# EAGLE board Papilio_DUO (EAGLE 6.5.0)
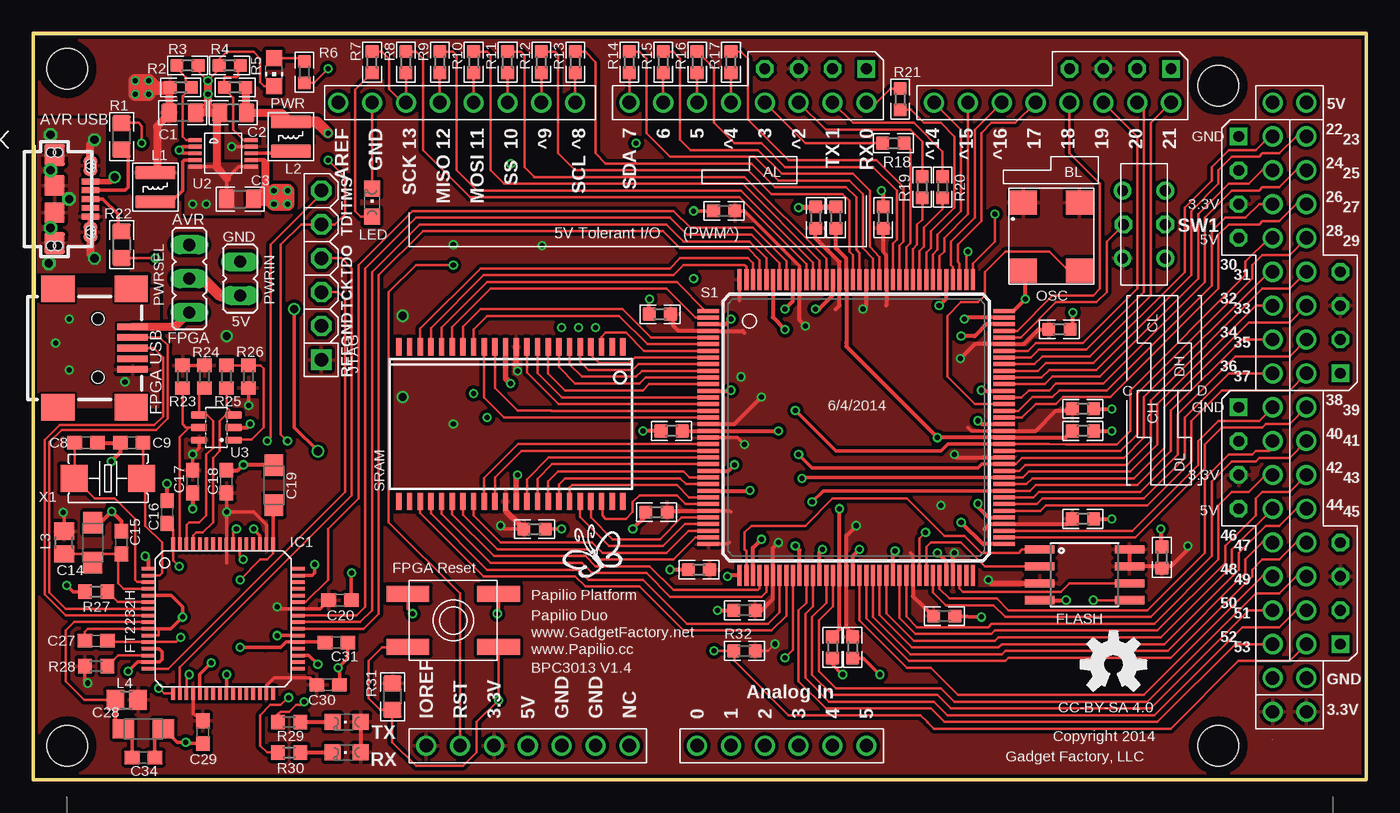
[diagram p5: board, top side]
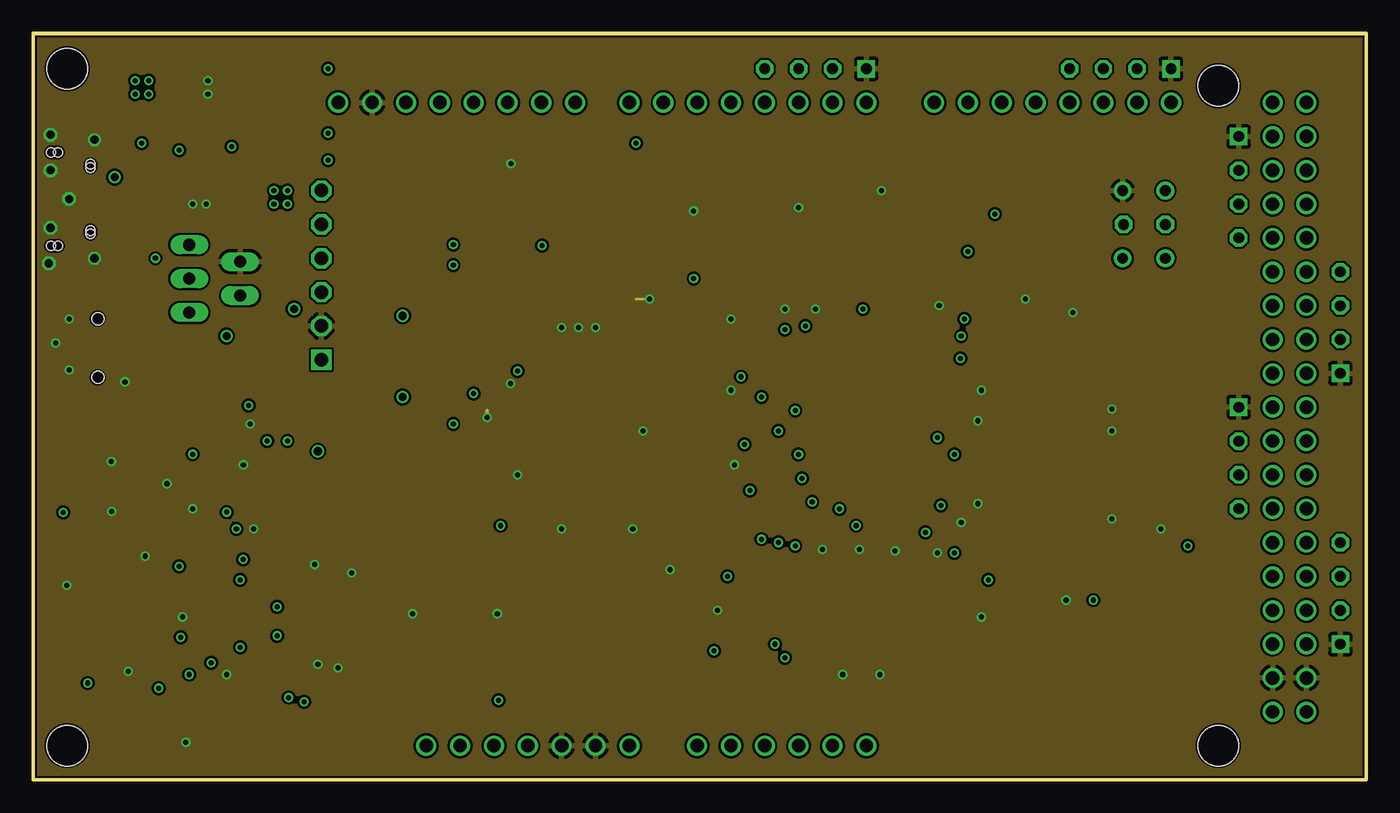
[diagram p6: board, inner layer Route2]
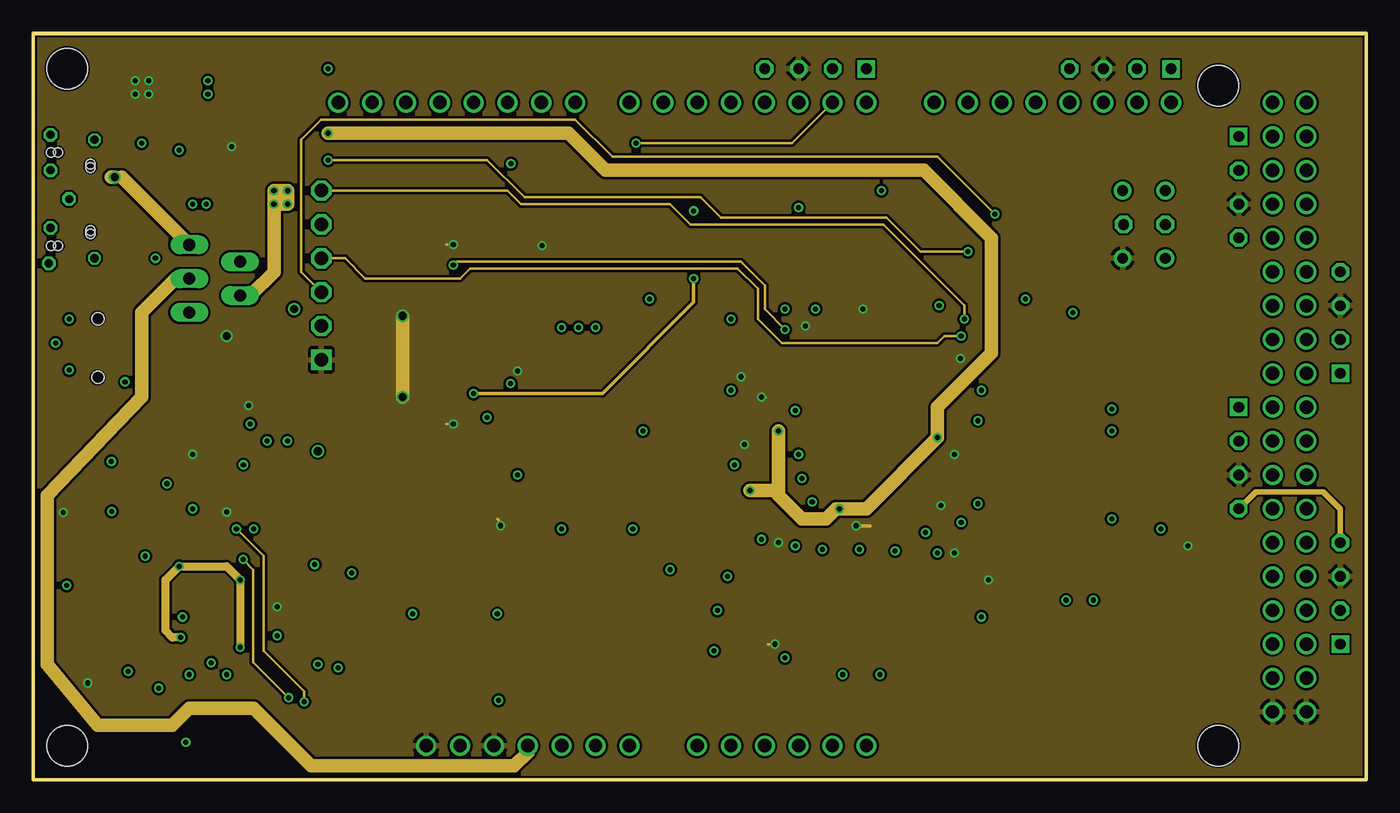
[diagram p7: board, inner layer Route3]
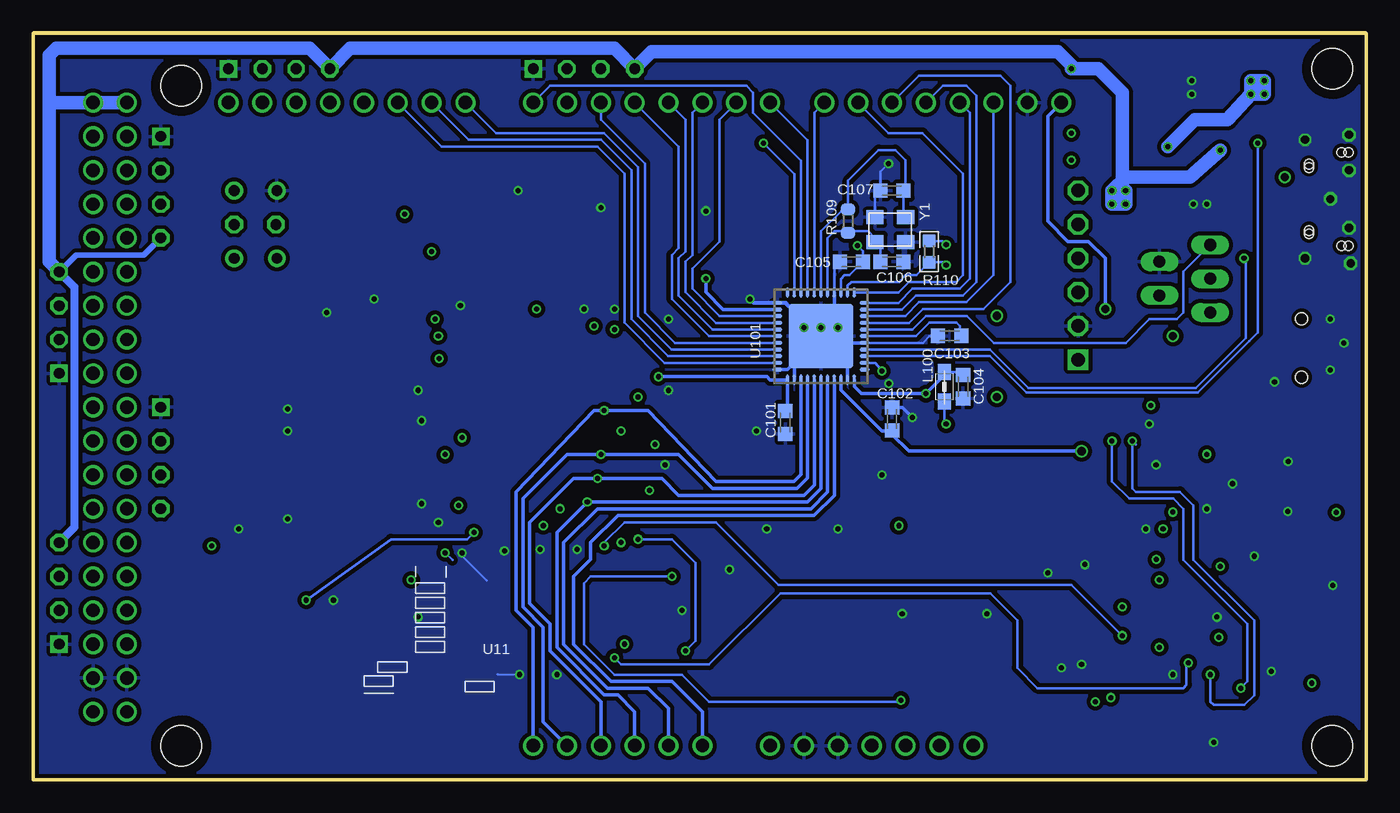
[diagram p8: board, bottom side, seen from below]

Size 100 x 56 mm. Coordinates in mm from the lower left corner, seen from the top.
Outline: 0,56 100,56 100,0 0,0 0,56
Outline: 0,56 56,56
Copper layers (1*2+3*16): Top 0.035mm / dielectric 1.5mm / Route2 0.035mm / dielectric 0.15mm / Route3 0.035mm / dielectric 0.2mm / Bottom 0.035mm
Design rules "hackvana *": minimum track width 6mil, minimum drill 0.3mm, track to track 6mil, track to pad 6mil, pad to pad 6mil, via to via 6mil, smd to smd 0mil, copper to edge 6mil, drill to drill 6mil, minimum pad ring 10mil, minimum via ring 6mil, stop-mask expansion 2mil, vias tented up to drill 100mil, thermal gap 10mil
Net classes: 0 default: width 0.178 mm, drill 0.381 mm, clearance 0.178 mm; 1 Power: width 0.254 mm, drill 0.381 mm, clearance 0.178 mm; 2 gnd: width 0.254 mm, drill 0.61 mm, clearance 0.254 mm; 3 usbvcc: width 0.254 mm, drill 0.61 mm, clearance 0.254 mm; 4 aref: width 0.254 mm, drill 0.61 mm, clearance 0.254 mm

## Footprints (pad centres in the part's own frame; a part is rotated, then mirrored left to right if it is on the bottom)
CON2_USB_MICRO_B_AT = smd 0.406 x 1.346: P1 -1.321,2.692; P2 -0.66,2.692; P3 0,2.692; P4 0.66,2.692; P5 1.321,2.692 | smd 1.651 x 1.549: S1 -3.302,0; S2 3.302,0 | smd 1.524 x 1.016: S3 -2.489,2.692; S4 2.489,2.692 | smd 1.524 x 1.524: S5 -1.016,0; S6 1.016,0 | hole 0.7: -3.505,0.254; -3.505,-0.254; 3.505,0.254; 3.505,-0.254; -2.616,2.692; -2.362,2.692; 2.362,2.692; 2.616,2.692
0805 = smd 1.2 x 1.4: 1 -1,0; 2 1,0
0603 = smd 1 x 1: 1 -0.8,0; 2 0.8,0
C603 = smd 1.1 x 1: 1 -0.85,0; 2 0.85,0
SMC_A = smd 1.6 x 1.4: + -1.5,0; - 1.5,0
C0603K = smd 1.05 x 1.08: 1 -0.875,0; 2 0.875,0
SO08-EIAJ = smd 0.61 x 2.21: 1 -1.905,-3.378; 2 -0.635,-3.378; 3 0.635,-3.378; 4 1.905,-3.378; 5 1.905,3.353; 6 0.635,3.353; 7 -0.635,3.353; 8 -1.905,3.353
CONN_USB_MINI-B = smd 2 x 2.5: BODY@1 -4.45,2.5; BODY@2 4.45,2.5; BODY@3 4.45,-3; BODY@4 -4.45,-3 | smd 0.5 x 2.3: D+ 0,2.6; D- -0.8,2.6; GND 1.6,2.6; ID 0.8,2.6; VUSB -1.6,2.6 | hole 0.9: -2.2,0; 2.2,0
LQFP64 = smd 1 x 0.27: 1 -5.6,3.75; 2 -5.6,3.25; 3 -5.6,2.75; 4 -5.6,2.25; 5 -5.6,1.75; 6 -5.6,1.25; 7 -5.6,0.75; 8 -5.6,0.25; 9 -5.6,-0.25; 10 -5.6,-0.75; 11 -5.6,-1.25; 12 -5.6,-1.75; 13 -5.6,-2.25; 14 -5.6,-2.75; 15 -5.6,-3.25; 16 -5.6,-3.75; 33 5.6,-3.75; 34 5.6,-3.25; 35 5.6,-2.75; 36 5.6,-2.25; 37 5.6,-1.75; 38 5.6,-1.25; 39 5.6,-0.75; 40 5.6,-0.25; 41 5.6,0.25; 42 5.6,0.75; 43 5.6,1.25; 44 5.6,1.75; 45 5.6,2.25; 46 5.6,2.75; 47 5.6,3.25; 48 5.6,3.75 | smd 0.27 x 1: 17 -3.75,-5.6; 18 -3.25,-5.6; 19 -2.75,-5.6; 20 -2.25,-5.6; 21 -1.75,-5.6; 22 -1.25,-5.6; 23 -0.75,-5.6; 24 -0.25,-5.6; 25 0.25,-5.6; 26 0.75,-5.6; 27 1.25,-5.6; 28 1.75,-5.6; 29 2.25,-5.6; 30 2.75,-5.6; 31 3.25,-5.6; 32 3.75,-5.6; 49 3.75,5.6; 50 3.25,5.6; 51 2.75,5.6; 52 2.25,5.6; 53 1.75,5.6; 54 1.25,5.6; 55 0.75,5.6; 56 0.25,5.6; 57 -0.25,5.6; 58 -0.75,5.6; 59 -1.25,5.6; 60 -1.75,5.6; 61 -2.25,5.6; 62 -2.75,5.6; 63 -3.25,5.6; 64 -3.75,5.6
VLS3015 = smd 3 x 1: 1 0,1.1; 2 0,-1.1
FB603 = smd 1.3 x 1.5: 1 -0.85,0; 2 0.85,0
0805' = smd 1.2 x 1: 1 -1.1,0; 2 1.1,0
CHIPLED_0805 = smd 1.2 x 1.2: A 0,-1.05; C 0,1.05
OSC1 = smd 1.8 x 2: 1@1 0,0; 2@2 5.08,0; 3@3 5.08,4.2; 4@4 0,4.2
CHIP-LED0805 = smd 1.2 x 1.2: A 0,-1.05; C 0,1.05
JP1 = drill 0.914 long: 1 0,-1.27; 2 0,1.27
JP2 = drill 0.914 long: 1 -2.54,0; 2 0,0; 3 2.54,0
R603 = smd 1 x 1.1: 1 -0.85,0; 2 0.85,0
R0603-ROUND = smd 0.898 x 1.1: 1 -0.889,0; 2 0.889,0
LED-805 = smd 1.2 x 1.2: A 0,-1.05; C 0,1.05
TQ144 = smd 1.6 x 0.3: 1 -11.1,8.75; 2 -11.1,8.25; 3 -11.1,7.75; 4 -11.1,7.25; 5 -11.1,6.75; 6 -11.1,6.25; 7 -11.1,5.75; 8 -11.1,5.25; 9 -11.1,4.75; 10 -11.1,4.25; 11 -11.1,3.75; 12 -11.1,3.25; 13 -11.1,2.75; 14 -11.1,2.25; 15 -11.1,1.75; 16 -11.1,1.25; 17 -11.1,0.75; 18 -11.1,0.25; 19 -11.1,-0.25; 20 -11.1,-0.75; 21 -11.1,-1.25; 22 -11.1,-1.75; 23 -11.1,-2.25; 24 -11.1,-2.75; 25 -11.1,-3.25; 26 -11.1,-3.75; 27 -11.1,-4.25; 28 -11.1,-4.75; 29 -11.1,-5.25; 30 -11.1,-5.75; 31 -11.1,-6.25; 32 -11.1,-6.75; 33 -11.1,-7.25; 34 -11.1,-7.75; 35 -11.1,-8.25; 36 -11.1,-8.75; 73 11.1,-8.75; 74 11.1,-8.25; 75 11.1,-7.75; 76 11.1,-7.25; 77 11.1,-6.75; 78 11.1,-6.25; 79 11.1,-5.75; 80 11.1,-5.25; 81 11.1,-4.75; 82 11.1,-4.25; 83 11.1,-3.75; 84 11.1,-3.25; 85 11.1,-2.75; 86 11.1,-2.25; 87 11.1,-1.75; 88 11.1,-1.25; 89 11.1,-0.75; 90 11.1,-0.25; 91 11.1,0.25; 92 11.1,0.75; 93 11.1,1.25; 94 11.1,1.75; 95 11.1,2.25; 96 11.1,2.75; 97 11.1,3.25; 98 11.1,3.75; 99 11.1,4.25; 100 11.1,4.75; 101 11.1,5.25; 102 11.1,5.75; 103 11.1,6.25; 104 11.1,6.75; 105 11.1,7.25; 106 11.1,7.75; 107 11.1,8.25; 108 11.1,8.75 | smd 0.3 x 1.6: 37 -8.75,-11.1; 38 -8.25,-11.1; 39 -7.75,-11.1; 40 -7.25,-11.1; 41 -6.75,-11.1; 42 -6.25,-11.1; 43 -5.75,-11.1; 44 -5.25,-11.1; 45 -4.75,-11.1; 46 -4.25,-11.1; 47 -3.75,-11.1; 48 -3.25,-11.1; 49 -2.75,-11.1; 50 -2.25,-11.1; 51 -1.75,-11.1; 52 -1.25,-11.1; 53 -0.75,-11.1; 54 -0.25,-11.1; 55 0.25,-11.1; 56 0.75,-11.1; 57 1.25,-11.1; 58 1.75,-11.1; 59 2.25,-11.1; 60 2.75,-11.1; 61 3.25,-11.1; 62 3.75,-11.1; 63 4.25,-11.1; 64 4.75,-11.1; 65 5.25,-11.1; 66 5.75,-11.1; 67 6.25,-11.1; 68 6.75,-11.1; 69 7.25,-11.1; 70 7.75,-11.1; 71 8.25,-11.1; 72 8.75,-11.1; 109 8.75,11.1; 110 8.25,11.1; 111 7.75,11.1; 112 7.25,11.1; 113 6.75,11.1; 114 6.25,11.1; 115 5.75,11.1; 116 5.25,11.1; 117 4.75,11.1; 118 4.25,11.1; 119 3.75,11.1; 120 3.25,11.1; 121 2.75,11.1; 122 2.25,11.1; 123 1.75,11.1; 124 1.25,11.1; 125 0.75,11.1; 126 0.25,11.1; 127 -0.25,11.1; 128 -0.75,11.1; 129 -1.25,11.1; 130 -1.75,11.1; 131 -2.25,11.1; 132 -2.75,11.1; 133 -3.25,11.1; 134 -3.75,11.1; 135 -4.25,11.1; 136 -4.75,11.1; 137 -5.25,11.1; 138 -5.75,11.1; 139 -6.25,11.1; 140 -6.75,11.1; 141 -7.25,11.1; 142 -7.75,11.1; 143 -8.25,11.1; 144 -8.75,11.1
TSOP44-II = smd 0.4 x 1.3: 1 -8.4,-5.8; 2 -7.6,-5.8; 3 -6.8,-5.8; 4 -6,-5.8; 5 -5.2,-5.8; 6 -4.4,-5.8; 7 -3.6,-5.8; 8 -2.8,-5.8; 9 -2,-5.8; 10 -1.2,-5.8; 11 -0.4,-5.8; 12 0.4,-5.8; 13 1.2,-5.8; 14 2,-5.8; 15 2.8,-5.8; 16 3.6,-5.8; 17 4.4,-5.8; 18 5.2,-5.8; 19 6,-5.8; 20 6.8,-5.8; 21 7.6,-5.8; 22 8.4,-5.8; 23 8.4,5.8; 24 7.6,5.8; 25 6.8,5.8; 26 6,5.8; 27 5.2,5.8; 28 4.4,5.8; 29 3.6,5.8; 30 2.8,5.8; 31 2,5.8; 32 1.2,5.8; 33 0.4,5.8; 34 -0.4,5.8; 35 -1.2,5.8; 36 -2,5.8; 37 -2.8,5.8; 38 -3.6,5.8; 39 -4.4,5.8; 40 -5.2,5.8; 41 -6,5.8; 42 -6.8,5.8; 43 -7.6,5.8; 44 -8.4,5.8
6P-2CH-2.54-9.1X3.5X3.2+2H = drill 0.813 pad 1.27: CH1A -2.54,-1.6; CH1B 2.54,-1.6; CH2A -2.54,1.6; CH2B 2.54,1.6 | drill 0.813 pad 1.27 octagon: COM1 0,-1.6; COM2 0,1.524
EVQ-Q2 = smd 3.2 x 1.2: A -3.4,-2; A' 3.4,-2; B -3.4,2; B' 3.4,2
ARDUINO_MEGA_SHIELD = drill 1 pad 1.422: 3.3V 50.8,26.67; 3V3@1 48.26,85.09; 3V3@2 48.26,87.63; 5V@0 50.8,29.21; 5V@1 2.54,85.09; 5V@2 2.54,87.63; A0 50.8,41.91; A1 50.8,44.45; A2 50.8,46.99; A3 50.8,49.53; A4 50.8,52.07; A5 50.8,54.61; AREF 2.54,14.986; D2 2.54,49.53; D3 2.54,46.99; D4 2.54,44.45; D5 2.54,41.91; D6 2.54,39.37; D7 2.54,36.83; D8 2.54,32.766; D9 2.54,30.226; D10 2.54,27.686; D11 2.54,25.146; D12 2.54,22.606; D13 2.54,20.066; D14 2.54,59.69; D15 2.54,62.23; D16 2.54,64.77; D17 2.54,67.31; D18 2.54,69.85; D19 2.54,72.39; D20 2.54,74.93; D21 2.54,77.47; D22 5.08,85.09; D23 5.08,87.63; D24 7.62,85.09; D25 7.62,87.63; D26 10.16,85.09; D27 10.16,87.63; D28 12.7,85.09; D29 12.7,87.63; D30 15.24,85.09; D31 15.24,87.63; D32 17.78,85.09; D33 17.78,87.63; D34 20.32,85.09; D35 20.32,87.63; D36 22.86,85.09; D37 22.86,87.63; D38 25.4,85.09; D39 25.4,87.63; D40 27.94,85.09; D41 27.94,87.63; D42 30.48,85.09; D43 30.48,87.63; D44 33.02,85.09; D45 33.02,87.63; D46 35.56,85.09; D47 35.56,87.63; D48 38.1,85.09; D49 38.1,87.63; D50 40.64,85.09; D51 40.64,87.63; D52 43.18,85.09; D53 43.18,87.63; GND@0 50.8,31.75; GND@1 50.8,34.29; GND@2 2.54,17.526; GND@3 45.72,85.09; GND@4 45.72,87.63; IOREF 50.8,21.59; RES 50.8,24.13; RX 2.54,54.61; TX 2.54,52.07; VIN 50.8,36.83
MSOP10 = smd 0.28 x 1: 1 -1,-2.1; 2 -0.5,-2.1; 3 0,-2.1; 4 0.5,-2.1; 5 1,-2.1; 6 1,2.1; 7 0.5,2.1; 8 0,2.1; 9 -0.5,2.1; 10 -1,2.1
SOT23-6 = smd 0.55 x 1.2: 1 -0.95,-1.3; 2 0,-1.3; 3 0.95,-1.3; 4 0.95,1.3; 5 0,1.3; 6 -0.95,1.3
QFN44ML7X7 = smd 0.75 x 0.275: 1 -3.275,2.5; 2 -3.275,2; 3 -3.275,1.5; 4 -3.275,1; 5 -3.275,0.5; 6 -3.275,0; 7 -3.275,-0.5; 8 -3.275,-1; 9 -3.275,-1.5; 10 -3.275,-2; 11 -3.275,-2.5; 23 3.275,-2.5; 24 3.275,-2; 25 3.275,-1.5; 26 3.275,-1; 27 3.275,-0.5; 28 3.275,0; 29 3.275,0.5; 30 3.275,1; 31 3.275,1.5; 32 3.275,2; 33 3.275,2.5 | smd 0.275 x 0.75: 12 -2.5,-3.275; 13 -2,-3.275; 14 -1.5,-3.275; 15 -1,-3.275; 16 -0.5,-3.275; 17 0,-3.275; 18 0.5,-3.275; 19 1,-3.275; 20 1.5,-3.275; 21 2,-3.275; 22 2.5,-3.275; 34 2.5,3.275; 35 2,3.275; 36 1.5,3.275; 37 1,3.275; 38 0.5,3.275; 39 0,3.275; 40 -0.5,3.275; 41 -1,3.275; 42 -1.5,3.275; 43 -2,3.275; 44 -2.5,3.275 | smd 4.826 x 4.826: EXP 0,0
JTAG = drill 1.016 octagon: JTAG_GND 10.16,0; JTAG_TCK 7.62,0; JTAG_TDI 2.54,0; JTAG_TDO 5.08,0; JTAG_TMS 0,0 | drill 1.016 square: JTAG_REF 12.7,0
STAND-OFF-TIGHT = hole 3.048: 0,0
POWER_NO_TEXT = drill 0.8 square: P1 0,3.81 | drill 0.8 octagon: P2 0,1.27; P3 0,-1.27; P4 0,-3.81
4X6 = smd 2.032 x 2.032: 1 -2.54,0; 2 2.54,0
CRYSTAL-3.2-2.5 = smd 1.3 x 1.05: 1 -1.15,-0.925; 2 1.15,-0.925; 3 1.15,0.925; 4 -1.15,0.925

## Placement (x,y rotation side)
AVRUSB  USB MICRO  [CON2_USB_MICRO_B_AT]  1.59,43.56 270 top
C1  22u/6V3  [0805]  11.19,50.04 180 top
C2  22u/6V3  [0805]  15,50.04 0 top
C3  10u/10V  [0805]  15.51,43.56 0 top
C4  .1uF  [0603]  47.01,34.92 180 top
C5  .1uF  [0603]  51.83,42.67 180 top
C6  .1uF  [0603]  58.69,42.16 90 top
C7  .1uF  [0603]  60.21,42.16 90 top
C8  27pF  [C603]  3.95,25.27 0 top
C9  27pF  [C603]  7.38,25.27 180 top
C10  .1uF  [0603]  47.9,26.16 180 top
C11  .1uF  [0603]  76.98,33.78 0 top
C12  .1uF  [0603]  78.76,27.81 0 top
C13  .1uF  [0603]  78.76,26.16 0 top
C14  4.7uF  [SMC_A]  4.46,17.78 90 top
C15  0.1uF  [C603]  6.62,17.78 90 top
C16  0.1uF  [C603]  10.05,20.07 90 top
C17  0.1uF  [C603]  11.95,22.35 270 top
C18  0.1uF  [C603]  14.49,22.35 90 top
C19  3.3uF  [SMC_A]  18.05,22.1 90 top
C20  0.1uF  [C603]  23,13.46 0 top
C21  .1uF  [0603]  37.61,18.8 0 top
C22  .1uF  [0603]  46.75,20.07 180 top
C23  .1uF  [0603]  49.93,15.75 180 top
C24  .1uF  [0603]  53.36,12.7 180 top
C25  .1uF  [0603]  78.76,19.56 0 top
C26  .1uF  [0603]  84.67,16.66 90 top
C27  0.1uF  [C603]  4.71,10.41 180 top
C28  4.7uF  [SMC_A]  8.27,3.81 0 top
C29  0.1uF  [C603]  12.72,3.56 270 top
C30  0.1uF  [C603]  22.11,7.11 0 top
C31  0.1uF  [C603]  22.75,10.29 0 top
C32  .1uF  [0603]  59.96,9.91 270 top
C33  .1uF  [0603]  61.48,9.91 270 top
C34  0.1uF  [C603]  8.27,1.65 0 top
C35  .1uF  [0603]  63.77,42.16 90 top
C36  .1uF  [0603]  68.34,12.27 0 top
C101  100n  [C0603K]  43.58,26.8 270 bottom
C102  100n  [C0603K]  35.58,27.05 270 bottom
C103  1uF  [C0603K]  31.24,33.29 180 bottom
C104  1uF  [C0603K]  30.24,29.46 270 bottom
C105  100n  [C0603K]  38.62,38.86 180 bottom
C106  22p  [C0603K]  35.58,38.86 180 bottom
C107  22p  [C0603K]  35.58,44.2 180 bottom
FLASH  FLASH-SPI-25XXSMD1  [SO08-EIAJ]  78.88,15.37 270 top
FPGAUSB  CONN_USB  [CONN_USB_MINI-B]  4.84,32.38 270 top
IC1  FT2232H  [LQFP64]  14.24,12.06 0 top
L1  3.3uH  [VLS3015]  9.16,44.45 180 top
L2  3.3uH  [VLS3015]  19.32,48.26 180 top
L3  [FB603]  2.3,17.78 90 top
L4  [FB603]  7,5.97 0 top
L100  MH2029-300Y  [0805']  31.64,29.46 90 bottom
LED  Yellow  [CHIPLED_0805]  25.42,43.31 0 top
OSC  [OSC1]  74.29,43.28 270 top
PWR  Green  [CHIP-LED0805]  18.05,53.09 180 top
PWRIN  [JP1]  15.51,37.59 0 top
PWRSEL  [JP2]  11.7,37.59 90 top
R1  22R  [0805]  6.62,48.26 90 top
R2  6K8 1%  [0603]  11.06,51.94 180 top
R3  1K5 1%  [0603]  11.57,53.59 180 top
R4  1K5 1%  [0603]  14.75,53.59 0 top
R5  1K5 1%  [0603]  15.13,51.94 0 top
R6  1K8  [0603]  20.34,53.09 270 top
R7  1K  [0603]  25.42,53.85 90 top
R8  390  [0603]  27.96,53.85 270 top
R9  390  [0603]  30.5,53.85 270 top
R10  390  [0603]  33.04,53.85 270 top
R11  390  [0603]  35.58,53.85 270 top
R12  390  [0603]  38.12,53.85 270 top
R13  390  [0603]  40.66,53.85 270 top
R14  390  [0603]  44.72,53.85 270 top
R15  390  [0603]  47.26,53.85 270 top
R16  390  [0603]  49.8,53.85 270 top
R17  390  [0603]  52.34,53.85 270 top
R18  390  [0603]  64.53,47.75 180 top
R19  390  [0603]  66.69,44.45 90 top
R20  390  [0603]  68.22,44.45 90 top
R21  390  [0603]  65.04,51.05 90 top
R22  22R  [0805]  6.62,40.13 270 top
R23  10k  [R603]  11.19,30.23 90 top
R24  10k  [R603]  12.84,30.23 90 top
R25  2.2k  [R603]  14.49,30.23 270 top
R26  10k  [R603]  16.14,30.23 270 top
R27  12k 1%  [R603]  4.71,14.1 0 top
R28  10k  [R603]  4.71,8.51 0 top
R29  470  [R603]  19.19,4.32 0 top
R30  470  [R603]  19.19,2.03 0 top
R31  47K  [0805]  26.94,6.22 90 top
R32  4.7K  [0603]  53.36,9.65 0 top
R109  1M  [R0603-ROUND]  38.88,41.91 270 bottom
R110  10K  [0603]  32.78,39.62 90 bottom
RX  [LED-805]  23.51,2.03 90 top
S1  6SLX9TQG144  [TQ144]  61.74,26.42 0 top
SRAM  [TSOP44-II]  35.83,26.67 180 top
SW1  SWITCH-2CH-6P-3010010P1  [6P-2CH-2.54-9.1X3.5X3.2+2H]  83.33,41.66 90 top
SW2  EVQQ2  [EVQ-Q2]  31.51,11.94 0 top
TX  [LED-805]  23.51,4.32 90 top
U1  ARDUINO_MEGA_SHIELD  [ARDUINO_MEGA_SHIELD]  7.89,53.34 270 top
U2  LTC3419EMS  [MSOP10]  14.24,46.99 270 top
U3  93C46B  [SOT23-6]  13.73,26.42 90 top
U101  ATMEGA32U4-XUMU  [QFN44ML7X7]  40.91,33.27 180 bottom
U$1  JTAG_XILINX  [JTAG]  21.61,44.2 270 top
U$2  [STAND-OFF-TIGHT]  2.54,53.34 0 top
U$3  [STAND-OFF-TIGHT]  2.54,2.54 0 top
U$4  [STAND-OFF-TIGHT]  88.9,2.54 0 top
U$5  [STAND-OFF-TIGHT]  88.9,52.07 0 top
U$7  [GADGETFACTORY_LOGO]  39.51,14.61 0 top
U$9  [OSHW-LOGO-M]  81.04,8.64 0 top
WING_POWER1  HEADER_FEMALE_4  [POWER_NO_TEXT]  58.69,53.34 270 top
WING_POWER2  HEADER_FEMALE_4  [POWER_NO_TEXT]  98.06,13.97 180 top
WING_POWER3  HEADER_FEMALE_4  [POWER_NO_TEXT]  98.06,34.29 180 top
WING_POWER4  HEADER_FEMALE_4  [POWER_NO_TEXT]  81.55,53.34 270 top
WING_POWER5  HEADER_FEMALE_4  [POWER_NO_TEXT]  90.44,44.45 0 top
WING_POWER6  HEADER_FEMALE_4  [POWER_NO_TEXT]  90.44,24.13 0 top
X1  12MHz  [4X6]  5.6,22.61 180 top
Y1  16MHz KX-7  [CRYSTAL-3.2-2.5]  35.7,41.27 180 bottom

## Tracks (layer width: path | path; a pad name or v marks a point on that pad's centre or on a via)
1.8V  (via drill 0.38)
  Top 0.203: v11.06,10.67 10.71,10.31 IC1.12 5.66,10.31 C27.1 | v10.94,16 10.49,16.45 IC1.64 10.49,18.77 C16.1 | 21.87,10.31 C31.1 | IC1.49 17.99,16.96 17.54,16.51 17.03,16.51 v15.51,14.99
  Top 0.254: IC1.49 17.99,20.54 C19.+ | v15.51,9.93 17.41,9.91 18.56,9.91 18.97,10.31 IC1.37 21.87,10.31
  Route3 0.61: v11.06,10.67 10.43,10.67 9.92,11.18 9.92,14.99 v10.94,16 14.49,16 v15.51,14.99 v15.51,9.93
1V2  (via drill 0.38)
  Top 0.203: 60.99,39.1 60.98,39.12 | 60.49,20.3 v60.47,20.32 | v55.89,26.17 v55.9,26.16 | 53.74,21.67 v53.76,21.69 | 67.85,25.67 v67.83,25.65 | 60.99,32.78 60.98,32.77
  Top 0.254: S1.19
  Top 0.305: 60.98,39.12 60.21,39.88 C7.1 | C10.1 S1.19 | 60.99,39.1 S1.128 60.99,32.78 60.99,32.5 v67.83,25.65 | 60.49,20.3 S1.52 60.49,11.3 C32.1 | S1.19 v55.89,26.17 | S1.28 53.74,21.67 | C13.1 77.44,25.67 S1.89 67.85,25.67
  Top 0.61: L2.2 18.64,50.04 C2.2 15.93,50.11 R5.2
  Top 0.813: L2.2 21.27,49.36 v22.11,48.51
  Route3 0.813: v60.47,20.32 60.21,20.32 | 55.9,21.34 55.9,21.59 55.79,21.69
  Route3 1.016: v22.11,48.51 40.15,48.51 42.94,45.72 66.82,45.72 71.9,40.64 71.9,32 67.83,27.94 v67.83,25.65 62.5,20.32 v60.47,20.32 | 60.21,20.32 59.45,19.56 57.67,19.56 55.9,21.34 | v55.9,26.16 55.9,21.59 | v53.76,21.69 55.79,21.69
3V3  (via drill 0.38, 0.6, 0.61)
  Top 0.203: C22.1 47.65,20.17 | 64.02,35.56 63.99,35.6 | 78.09,27.69 C12.1 77.83,27.69 | FLASH.8 82.22,16.02 | 35.94,19.67 35.92,19.67 | 35.45,20.85 SRAM.33 | 48.02,34.71 C4.1 | R32.2 55.13,9.65 v55.64,10.16 | 14.49,16.26 | 14.49,18.29 14.49,18.28 IC1.56 | v14.49,20.06 v14.49,20.07
  Top 0.254: S1.122 64.02,37.55 | S1.18 52.34,26.67 | S1.20 52.84,25.67 v53.36,25.15 | S1.31 52.24,20.17 52.34,20.07 | S1.63 65.99,16.83 65.8,17.02 | S1.90 70.37,26.17 70.12,26.42 | C5.1 53.36,42.67 57.49,38.54 S1.135 | U2.9 v14.88,47.5 | v18.3,12.95 18.44,12.81 IC1.42 21.51,12.81 C20.1 | R26.2 v16.14,28.07 | IC1.31 17.49,7.06 18.05,7.62 20.76,7.62 C30.1 | R28.1 3.87,7.45 v4.08,7.24 | L3.2 2.3,19.99 v2.25,20.04 | C18.1 v14.49,20.07 16.53,20.07 17.49,19.1 IC1.50 | U3.6 12.43,24.89 v11.95,24.41 C17.1 | IC1.20 11.99,4.95 C29.1 | C21.1 35.32,18.8 v35.07,19.05 | 14.49,16.26 IC1.56 | 14.49,18.28 v14.49,20.06 | R23.2 R24.2 | S1.144 52.99,35.95 52.98,35.94 | S1.36 52.1,17.67 52.21,17.78
  Top 0.305: 53.36,33.53 53.22,33.67 S1.4 48.39,33.67 48.02,34.04 48.02,34.71 | 71.39,18.8 71.76,19.17 S1.76 77.59,19.17 C25.1 | C6.1 58.69,40.64 60.49,38.84 S1.129 60.49,35.58 60.21,35.31 | 47.65,20.17 S1.31 | C24.1 54.63,12.7 55.49,13.56 S1.42 55.49,17.37 v55.9,17.78 | S1.86 69.32,24.17 v69.1,24.38 | FLASH.8 FLASH.7 | S1.90 75.2,26.17 76.72,27.69 77.83,27.69 | C33.1 61.48,10.92 60.99,11.42 S1.53 60.99,18.3 v61.74,19.05 | S1.69 68.99,16.9 v69.1,17.02 | S1.135 57.49,34.48 v57.93,34.04 | S1.125 62.49,35.55 v62.25,35.31 | TX.A RX.A | v69.56,31.6 70.63,32.67 S1.103 74.3,32.67 75.42,33.78 C11.1 | S1.18 52.59,26.67 v54.63,28.7 | C35.1 63.77,39.62 63.99,39.33 S1.122 63.99,35.6 | S1.63 65.99,13.75 C36.1 | 82.22,16.02 84.52,16.02 C26.1 84.81,16 85.36,16 86.63,17.27 v86.63,17.53
  Top 0.406: C21.1 35.94,19.67 | v71.64,14.99 71.9,14.73 FLASH.3 | 35.92,19.67 35.45,20.14 35.45,20.85 | SRAM.11 36.23,30.7 v36.34,30.66
  Top 0.61: R2.2 10.19,51.87 C1.2 9.29,49.02 9.29,45.68 L1.2
  Top 1.016: 10.19,51.87 9.23,51.87 v8.65,52.45 v7.64,52.45 v7.64,51.44 v8.65,51.44
  Route3 0.178: v31.51,26.67 31,26.67
  Route3 0.203: v35.07,19.05 35.07,19.3 34.81,19.56 | v31.51,40.13 31,40.13 | v55.64,10.16 55.13,10.16 | v55.9,17.78 56.15,17.78
  Route3 0.254: v61.74,19.05 62.75,19.05
  Route3 0.305: v54.63,28.7 54.88,28.7
  Route3 1.016: v27.7,28.7 v27.7,34.8
  Bottom 0.178: L100.1 31.64,26.8 v31.51,26.67
  Bottom 0.203: U101.2 36.8,31.27 v36.34,30.66 | R110.2 31.8,40.42 v31.51,40.13 | U101.14 39.41,37.57 39.13,37.85 38.77,37.85 C105.1 37.75,39.64 v38.17,40.06 | 68.56,16.47 v69.1,17.02
  Bottom 0.254: v53.1,30.23 44.97,30.23 44.75,30 U101.34 43.41,27.84 C101.1
  Bottom 1.016: v8.65,51.44 v7.64,51.44 v7.64,52.45 v8.65,52.45 v8.65,51.44 | v14.88,47.5 12.84,49.53 10.43,49.53 v8.65,51.44
  other vias: 68.09,20.57 14.49,33.27
  pour Top (isolate 0.254, rank 3): 0,56 0,0 100,0 100,56
  pour Route3: 0,56 100,56 100,0 0,0
5V0  (via drill 0.38)
  Top 0.203: R6.2 21.06,52.29 v22.11,53.34
  Top 0.254: U2.3 11.19,46.99 v10.94,47.24 11.18,47.49 U2.2
  Top 0.305: U2.7 17.29,46.48 17.41,46.36 17.41,46.23
  Top 0.61: 17.41,46.23 17.41,44.34 C3.2
  Top 0.813: 18.05,43.69 18.56,44.2 | PWRSEL.2 12.72,37.59 13.99,36.32 PWRIN.1
  Top 1.016: C3.2 17.67,43.56 v18.05,43.18 | v18.05,43.18 v18.05,44.2 18.56,44.2 v19.07,44.2 v19.07,43.18 18.81,43.18 | 18.81,43.18 v18.05,43.18 | 18.68,43.56 18.81,43.18
  Route3 0.406: WING_POWER2.P4 98.06,20.32 96.79,21.59 91.71,21.59 WING_POWER6.P4
  Route3 1.016: PWRIN.1 16.27,36.32 18.05,38.1 v18.05,43.18 | U1.5V@0 37.1,2.03 36.08,1.02 20.84,1.02 16.53,5.33 11.7,5.33 10.43,4.06 4.84,4.06 1.03,8.64 1.03,21.34 8.14,28.7 8.14,35.05 10.68,37.59 PWRSEL.2 | v18.05,43.18 v18.05,44.2 v19.07,44.2 v19.07,43.18 v18.05,43.18
  Bottom 0.406: WING_POWER3.P4 96.79,39.37 91.71,39.37 WING_POWER5.P4
  Bottom 0.61: 18.3,44.45 v18.05,44.2 | WING_POWER3.P4 96.92,36.96 96.92,18.92 WING_POWER2.P4
  Bottom 0.813: v22.11,53.34 22.11,53.59
  Bottom 1.016: v19.07,44.2 18.05,45.21 13.22,45.21 v10.94,47.24 | v19.07,44.2 v19.07,43.18 v18.05,43.18 v18.05,44.2 v19.07,44.2 | v22.11,53.34 20.08,53.34 18.3,51.56 18.3,44.45 | U1.5V@1 U1.5V@2 98.82,50.8 | 22.11,53.59 23.13,54.61 53.61,54.61 WING_POWER1.P4 56.4,54.86 76.22,54.86 WING_POWER4.P4 79.26,54.86 98.3,54.86 98.82,54.34 98.82,50.8 | 98.82,50.8 98.82,38.86 WING_POWER3.P4
5V_ARDUINO  (via drill 0.61)
  Top 0.406: AVRUSB.P1 5.78,44.88 v6.11,45.21
  Route3 0.61: v6.11,45.21 6.62,45.21
  Route3 1.016: 5.86,45.21 v6.11,45.21 | 6.62,45.21 PWRSEL.3
  Bottom 0.203: U101.7 34.04,33.77 33.02,34.8 29.97,34.8 27.94,32.77 18.03,32.77 16.26,34.54 14.22,34.54 13.72,35.05 13.72,38.12 PWRSEL.3
5V_FT2232
  Top 0.61: FPGAUSB.VUSB 10.63,33.98 PWRSEL.1
!CS
  Top 0.203: S1.12 46.19,29.67 45.74,29.21 39.89,29.21 38.63,30.47 SRAM.8
!OE
  Top 0.203: S1.26 49.23,22.67 48.78,23.11 39.39,23.11 38.63,22.36 SRAM.37
!RESET
  Top 0.203: IC1.14 6.37,9.31 R28.2
!WE
  Top 0.203: S1.6 46.09,32.67 43.96,34.8 34.05,34.8 33.03,33.78 SRAM.15
A0
  Top 0.203: S1.7 45.83,32.17 44.47,33.53 42.94,33.53 42.63,33.22 SRAM.3
A1
  Top 0.203: S1.8 45.14,31.67 44.72,31.24 42.43,31.24 41.83,31.85 SRAM.4
A2
  Top 0.203: S1.9 45.41,31.17 44.97,30.73 41.67,30.73 41.03,31.38 SRAM.5
A3
  Top 0.203: S1.10 45.67,30.67 45.23,30.23 41.16,30.23 40.23,31.16 SRAM.6
A4
  Top 0.203: S1.11 45.93,30.17 45.48,29.72 40.66,29.72 39.43,30.94 SRAM.7
A5
  Top 0.203: S1.5 46.35,33.17 44.21,35.31 33.54,35.31 32.23,33.99 SRAM.16
A6
  Top 0.203: SRAM.17 31.43,33.95 34.31,36.83 47.51,36.83 49.68,34.67 S1.2
A7
  Top 0.203: S1.1 50.45,35.17 48.28,37.34 34.05,37.34 30.63,33.92 SRAM.18
A8
  Top 0.203: SRAM.19 29.83,33.88 33.8,37.85 48.02,37.85 48.78,38.61 53.36,38.61 53.49,38.48 S1.143
A9
  Top 0.203: S1.142 53.99,38.74 53.61,39.12 48.53,39.12 47.77,38.35 33.54,38.35 29.03,33.84 SRAM.20
A10
  Top 0.203: S1.43 55.99,12.54 55.13,11.68 49.04,11.68 45.74,14.99 41.67,14.99 40.91,15.75 34.05,15.75 29.83,19.97 SRAM.26
A11
  Top 0.203: S1.41 54.99,14.08 54.63,13.72 47.77,13.72 45.99,15.49 41.93,15.49 41.16,16.26 34.31,16.26 30.63,19.93 SRAM.27
A12
  Top 0.203: S1.40 54.49,14.34 54.37,14.22 48.02,14.22 46.24,16 42.18,16 41.42,16.76 34.56,16.76 31.43,19.89 SRAM.28
A13
  Top 0.203: S1.35 49.68,18.17 48.02,16.51 42.43,16.51 41.67,17.27 34.81,17.27 32.23,19.86 SRAM.29
A14
  Top 0.203: S1.34 49.16,18.67 47.51,17.02 42.69,17.02 41.93,17.78 35.07,17.78 33.03,19.82 SRAM.30
A15
  Top 0.203: S1.27 48.97,22.17 48.53,22.61 39.89,22.61 39.43,22.14 SRAM.38
A16
  Top 0.203: S1.29 49.21,21.17 48.28,22.1 40.4,22.1 40.23,21.93 SRAM.39
A17
  Top 0.203: S1.33 48.9,19.17 47.26,17.53 43.2,17.53 41.03,19.69 SRAM.40
A18
  Top 0.203: S1.32 48.64,19.67 47.01,18.03 43.45,18.03 41.83,19.65 SRAM.41
A19
  Top 0.203: S1.44 56.49,12.28 55.39,11.18 48.78,11.18 45.48,14.48 41.42,14.48 40.66,15.24 33.8,15.24 29.03,20.01 SRAM.25
A20
  Top 0.203: S1.30 48.95,20.67 48.28,21.34 45.48,21.34 44.97,20.83 44.97,20.07 44.47,19.56 42.94,19.56 42.69,19.81 42.69,20.81 SRAM.42
AD0-JTAG_TCK  (via drill 0.38)
  Top 0.203: IC1.16 10.11,8.31 23.38,21.59 23.38,36.07 22.88,36.58 U$1.JTAG_TCK | S1.109 70.49,38.72 72.15,40.39 v72.15,42.42
  Route3 0.203: v72.15,42.42 67.83,46.74 43.45,46.74 40.66,49.53 21.61,49.53 20.08,48.01 20.08,38.1 U$1.JTAG_TCK
AD1-JTAG_TDI  (via drill 0.38)
  Top 0.203: IC1.17 9.81,6.46 v9.41,6.86 | S1.110 69.99,39.5 v70.12,39.62 | v19.07,25.4 18.56,25.91 18.56,40.13 20.08,41.66 U$1.JTAG_TDI 22.62,41.66 23.38,42.42 23.38,45.21 v22.11,46.48
  Route3 0.203: v70.12,39.62 66.56,39.62 64.02,42.16 51.58,42.16 50.05,43.69 36.85,43.69 34.05,46.48 v22.11,46.48
  Bottom 0.203: v9.41,6.86 8.91,7.37 8.91,11.68 13.72,16.49 13.72,20.32 14.48,21.08 17.78,21.08 19.07,22.37 v19.07,25.4
AD2-JTAG_TDO  (via drill 0.38)
  Top 0.203: IC1.18 10.99,8.43 23.89,21.34 23.89,38.35 23.13,39.12 U$1.JTAG_TDO
  Top 0.305: S1.106 71.52,34.17 70.63,33.27 v69.61,33.27
  Route3 0.203: U$1.JTAG_TDO 23.38,39.12 24.91,37.59 32.02,37.59 32.78,38.35 52.85,38.35 54.37,36.83 54.37,34.54 56.15,32.77 67.83,32.77 68.34,33.27 v69.61,33.27
AD3-JTAG_TMS  (via drill 0.38)
  Top 0.203: v17.54,25.4 17.8,25.65 17.8,40.13 21.61,43.94 U$1.JTAG_TMS | IC1.19 11.49,7.68 v11.68,7.87
  Top 0.305: S1.107 69.99,34.67 v69.87,34.54
  Route3 0.203: v69.87,34.54 69.87,35.56 63.77,41.66 49.29,41.66 47.77,43.18 36.59,43.18 35.58,44.2 U$1.JTAG_TMS
  Bottom 0.203: 17.29,25.15 v17.54,25.4 17.54,21.86 17.27,21.59 13.97,21.59 12.95,20.57 12.95,16.49 8.4,11.94 8.4,6.33 9.14,5.59 11.43,5.59 11.68,5.84 v11.68,7.87
AD4-DTR  (via drill 0.38)
  Top 0.203: S1.45 56.99,9.73 v56.4,9.14
  Top 0.254: IC1.21 12.49,7.9 v13.35,8.76
  Bottom 0.203: v56.4,9.14 55.9,8.64 49.29,8.64 43.96,13.97 28.21,13.97 26.18,11.94 26.18,8.38 24.65,6.86 13.73,6.86 13.48,7.11 13.48,8.64 v13.35,8.76
ARD_RESET  (via drill 0.38)
  Top 0.203: U1.RES 32.02,13.95 26.67,19.3 26.67,36.58 28.7,38.61 v31.51,38.61
  Top 0.305: v56.4,33.78 55.49,34.7 S1.139
  Route3 0.203: v56.4,33.78 54.88,35.31 54.88,37.08 53.1,38.86 31.77,38.86 v31.51,38.61
  Bottom 0.203: U101.13 38.91,37.05 38.62,37.34 35.07,37.34 34.56,37.85 33.76,37.85 R110.1 31.73,38.82 v31.51,38.61
AREF  (via drill 0.61)
  Top 0.254: v19.57,35.31 19.57,26.42 v21.35,24.64
  Bottom 0.254: U101.42 39.41,29.23 36.34,26.16 35.59,26.16 C102.2 35.58,25.91 34.31,24.64 v21.35,24.64 | U1.AREF 23.89,49.78 23.89,41.91 22.37,40.39 20.84,40.39 19.57,39.12 v19.57,35.31
ATMEGA_A0
  Bottom 0.254: U101.41 39.91,21.32 41.42,19.81 56.15,19.81 58.18,17.78 58.18,16.51 59.45,15.24 59.45,10.16 56.66,7.37 52.09,7.37 49.8,5.08 U1.A0
ATMEGA_A1
  Bottom 0.254: U101.40 40.41,21.58 41.67,20.32 57.67,20.32 60.21,17.78 60.21,10.16 56.91,6.86 53.86,6.86 52.34,5.33 U1.A1
ATMEGA_D0/RX
  Top 0.203: R21.2 64.32,51.85 63.26,50.8 U1.RX
  Bottom 0.203: U101.20 42.41,46.46 45.99,50.04 45.99,51.56 46.5,52.07 61.23,52.07 U1.RX
ATMEGA_D1/TX  (via drill 0.38)
  Top 0.203: U1.TX 61.48,49.28 66.06,49.28 68.22,47.12 R20.2
  Route3 0.203: v45.23,47.75 56.91,47.75 U1.TX
  Bottom 0.203: U101.21 42.91,45.43 v45.23,47.75
ATMEGA_D2
  Top 0.203: U1.D2 59.45,48.77 65.8,48.77 66.69,47.88 R19.2
  Bottom 0.203: U101.29 51.84,32.77 54.12,35.05 54.12,46.23 57.42,49.53 U1.D2
ATMEGA_D3
  Top 0.203: U1.D3 57.93,47.75 R18.2
  Bottom 0.203: U101.28 49.29,33.27 52.09,36.07 52.09,39.37 51.58,39.88 51.58,47.5 U1.D3
ATMEGA_D4
  Top 0.203: U1.D4 R17.2
  Bottom 0.203: U101.27 49.03,33.77 51.58,36.32 51.58,39.12 51.07,39.62 51.07,49.53 U1.D4
ATMEGA_D5*
  Top 0.203: U1.D5 R16.2
  Bottom 0.203: U101.26 48.77,34.27 51.07,36.58 51.07,38.86 50.56,39.37 50.56,50.04 U1.D5
ATMEGA_D6*
  Top 0.203: U1.D6 R15.2
  Bottom 0.203: U101.25 48.51,34.77 50.56,36.83 50.56,38.35 48.53,40.39 48.53,49.53 U1.D6
ATMEGA_D7
  Top 0.203: U1.D7 R14.2
  Bottom 0.203: U101.19 41.91,47.99 U1.D7
ATMEGA_IO8
  Top 0.203: U1.D8 R13.2
  Bottom 0.203: U101.18 41.41,50.05 U1.D8
ATMEGA_IO9*
  Top 0.203: U1.D9 R12.2
  Bottom 0.203: U101.12 35.09,36.55 34.31,37.34 30.75,37.34 30.24,37.85 30.24,45.47 33.29,48.51 35.83,48.51 U1.D9
ATMEGA_IO10*
  Top 0.203: U1.D10 R11.2
  Bottom 0.203: U1.D10 33.54,52.83 27.45,52.83 26.69,52.07 26.69,37.34 28.72,35.31 33.27,35.31 34.31,34.27 U101.8
ATMEGA_IO11*
  Top 0.203: U1.D11 R10.2
  Bottom 0.203: U101.10 34.85,35.27 33.8,36.32 30.24,36.32 29.23,37.34 29.23,51.31 29.99,52.07 31.77,52.07 U1.D11
ATMEGA_IO12
  Top 0.203: U1.D12 R9.2
  Bottom 0.203: U101.11 35.11,35.77 34.05,36.83 30.5,36.83 29.73,37.59 29.73,50.04 U1.D12
ATMEGA_IO13*
  Top 0.203: R8.2 U1.D13 27.7,50.8 26.69,51.82 26.69,54.1 26.18,54.61 25.45,54.61 R7.2
  Bottom 0.203: U101.9 34.58,34.77 33.54,35.81 29.99,35.81 27.96,37.85 U1.D13
AVCC  (via drill 0.38)
  Route3 0.254: v49.55,37.59 49.55,35.81 42.69,28.96 v33.04,28.96
  Bottom 0.178: L100.2 30.47,30.56 C104.1
  Bottom 0.254: U101.24 48.24,35.27 49.55,36.58 v49.55,37.59 | U101.44 38.41,29.5 37.86,28.96 v33.04,28.96 31.64,30.35 L100.2
AVRUSB_N  (via drill 0.38)
  Top 0.178: 8.14,47.75 v8.13,47.75 8.13,49.04 7.89,49.28 6.64,49.28 R1.2
  Bottom 0.178: U101.3 28.23,31.77 25.49,29.03 12.64,29.03 8.78,32.89 8.14,33.53 8.14,47.26 v8.13,47.75
AVRUSB_P  (via drill 0.38)
  Top 0.178: v9.16,39.12 6.64,39.12 R22.2
  Bottom 0.178: U101.4 28.23,32.27 25.34,29.39 12.79,29.39 9.03,33.15 9.03,38.99 v9.16,39.12
BC3  (via drill 0.38)
  Top 0.203: IC1.54 15.49,16.77 v15.75,16.51 | v19.15,6.15 19.1,6.15 18.54,5.59 17.78,5.59 17.02,4.83 17.02,2.54 17.53,2.03 R30.1
  Route3 0.203: v15.75,16.51 16.51,15.75 16.51,8.79 v19.15,6.15
BC4  (via drill 0.38)
  Top 0.203: IC1.55 14.99,18.55 v15.24,18.8 | R29.1 18.34,4.88 18.54,5.08 19.2,5.08 19.71,5.59 20.07,5.59 v20.32,5.84
  Route3 0.203: v20.32,5.84 20.32,6.6 17.27,9.65 17.27,16.76 v15.24,18.8
BD0_TXD/MPSSE_TCK  (via drill 0.38)
  Top 0.203: 18.32,10.81 v18.3,10.79
  Top 0.254: IC1.38 18.32,10.81
  Top 0.305: S1.46 57.49,17.2 v57.17,17.53
  Bottom 0.203: v18.3,10.79 22.11,14.61 44.09,14.61 48.78,19.3 55.64,19.3 57.17,17.78 v57.17,17.53
BD1_RXD/MPSSE_TDI
  Top 0.203: IC1.39 24.79,11.31 25.92,12.45 25.92,37.85 29.23,41.15 47.26,41.15 48.53,39.88 53.61,39.88 54.49,39 S1.141
BD2_MPSSE_TDO
  Top 0.203: IC1.40 24.53,11.81 25.42,12.7 25.42,38.1 28.97,41.66 47.51,41.66 48.78,40.39 53.74,40.39 54.99,39.13 S1.140
BD3_MPSSE_TMS
  Top 0.203: S1.138 55.99,38.77 53.86,40.89 49.04,40.89 47.77,42.16 28.72,42.16 24.91,38.35 24.91,12.95 24.27,12.31 IC1.41
BD4-DTR
  Top 0.203: S1.137 56.49,38.91 53.99,41.4 49.29,41.4 48.02,42.67 28.46,42.67 24.4,38.61 24.4,21.08 22.11,18.8 22.11,14.99 20.44,13.31 IC1.43
D0
  Top 0.203: S1.14 39.68,28.67 37.83,30.51 SRAM.9
D1
  Top 0.203: S1.15 39.41,28.17 37.03,30.55 SRAM.10
D2
  Top 0.203: S1.16 38.9,27.67 38.88,27.69 36.32,27.69 34.63,29.38 SRAM.13
D3
  Top 0.203: S1.17 37.11,27.17 37.1,27.18 35.31,27.18 33.83,28.65 SRAM.14
D4
  Top 0.203: SRAM.31 33.83,22.64 36.36,25.17 S1.21
D5
  Top 0.203: SRAM.32 34.63,22.68 36.62,24.67 S1.22
D6
  Top 0.203: SRAM.35 37.03,22.54 38.66,24.17 S1.23
D7
  Top 0.203: SRAM.36 37.83,22.57 38.92,23.67 S1.24
D+
  Top 0.254: AVRUSB.P3 5.22,43.56 6.37,42.42 6.37,41.39 R22.1
D-
  Top 0.254: AVRUSB.P2 6.9,44.22 7.13,44.45 7.13,46.75 R1.1
EECLK
  Top 0.203: IC1.62 11.49,19.09 11.7,19.3 12.46,19.3 12.97,19.81 12.97,24.38 13.48,24.89 13.48,26.92 13.04,27.37 U3.4 12.43,28.96 R24.1
EECS
  Top 0.178: IC1.63 10.99,25.71 11.7,26.42
  Top 0.203: U3.5 11.7,26.42 11.45,26.42 11.19,26.67 R23.1
EEDATA
  Top 0.203: R25.2 14.49,27.9 U3.3 14.43,27.37 13.99,26.92 13.99,24.64 13.48,24.13 13.48,19.3 12.72,18.54 12.21,18.54 11.99,18.32 IC1.61
FB_1V2
  Top 0.203: U2.10 15.78,47.99 15,48.77 15,51.18 14.33,51.85 R5.1 14.33,52.67 14.37,52.7 15.26,52.7 15.38,52.83 15.38,53.43 R4.2
FB_3V3
  Top 0.203: U2.1 11.46,47.99 11.19,48.26 11.19,51.27 R2.1 11.45,52.36 11.45,52.7 10.77,53.38 R3.2
FLASH_CS
  Top 0.203: FLASH.1 74.18,17.27 73.93,17.02 71.14,17.02 69.87,18.29 68.34,18.29 65.55,21.08 59.96,21.08 57.93,19.05 53.86,19.05 53.36,18.54 53.36,17.27 53.49,17.14 S1.38
FLASH_SCK
  Top 0.203: S1.70 69.49,14.35 69.74,14.1 77.11,14.1 77.74,14.73 FLASH.6
FLASH_SI  (via drill 0.38)
  Top 0.203: v79.52,13.46 FLASH.5 | S1.64 66.49,18.11 v66.94,18.54
  Bottom 0.203: v79.52,13.46 73.17,18.03 67.45,18.03 v66.94,18.54
FLASH_SO
  Top 0.203: S1.65 66.99,17.44 67.33,17.78 69.61,17.78 71.39,16 FLASH.2
FTUSB_N
  Top 0.178: IC1.7 2.44,12.81 1.21,14.04 1.21,25.33 2.12,26.24 9.22,26.24 10.08,27.1 10.08,32.59 9.49,33.19 FPGAUSB.D-
FTUSB_P
  Top 0.178: IC1.8 2.44,12.31 0.85,13.9 0.85,25.47 1.97,26.59 9.07,26.59 9.73,27.25 9.73,31.67 9.02,32.38 FPGAUSB.D+
GND  (via drill 0.38, 0.61, 0.61 pad 1.02)
  Top 0.203: 71.18,29.17 v71.14,29.21 | 52.3,29.17 v52.34,29.21 | 84.65,17.58 C26.2 | C32.2 59.97,9.16 | R3.1 12.37,53.17 v13.1,52.45 13.95,53.3 R4.1 13.99,53.63 13.99,54.1 14.49,54.61 16.53,54.61 17.03,54.1 17.03,52.32 17.32,52.04 PWR.C | v14.49,7.87 | C27.2 3.87,11.09 4.08,11.3 8.63,11.3 IC1.10 | C14.- 5.05,19.28 | 22.96,8.29 v22.88,8.38 | 23.85,15.46 v23.89,15.49 | 15.79,23.6 v15.76,23.62 | C22.2 45.95,19.77 | C11.2 77.99,33.78 | OSC.2@2 74.41,38.08 | LED.C U1.GND@2 | C36.2 69.1,12.19 | IC1.11 9.41,10.81 9.41,11.31 | C28.- 9.16,3.81
  Top 0.254: v49.55,42.67 C5.2 | C21.2 v39.64,18.8 | U2.6 15.4,45.99 14.51,45.1 C3.1 | 13.75,45.99 U2.5 | IC1.47 20.92,15.31 21.1,15.49 v21.1,16.13 | IC1.25 v14.49,7.87 | IC1.13 9.45,9.81 9.67,9.6 9.67,9.02 9.47,8.81 IC1.15 7.82,8.81 v7.13,8.13 | IC1.51 16.99,18.33 v16.53,18.8 | IC1.10 9.41,11.31 10.31,11.31 v11.19,12.19 11.19,12.95 10.33,13.81 IC1.5 | R27.1 2.99,14.1 v2.5,14.58 | C30.2 22.96,8.29 | IC1.35 20.67,9.31 v21.35,8.64 | C31.2 23.6,9.11 v22.88,8.38 | C20.2 23.85,15.46 | SW2.B 28.11,12.8 v28.46,12.45 | SW2.B' 34.91,12.54 v34.81,12.45 | 59.97,9.16 59.97,8.9 59.96,8.64 v60.72,7.87 | C33.2 62.28,9.11 v63.52,7.87 | C29.2 11.45,2.71 v11.45,2.79 10.79,2.79 C28.- | C34.2 9.12,3.77 9.16,3.81
  Top 0.305: S1.113 68.49,36.09 v67.96,35.56 | 71.18,29.17 S1.96 | S1.91 71.14,26.67 v70.88,26.92 | S1.60 64.49,16.97 v64.66,17.14 | S1.13 52.3,29.17 | S1.136 56.99,35.89 v56.4,35.31 | C10.2 v45.74,26.16 | C23.2 v47.77,15.75 | C25.2 v80.92,19.56 | C13.2 v80.92,26.16 | C12.2 v80.92,27.81 | v51.32,12.7 C24.2 | FLASH.4 v77.49,13.46 | S1.54 61.49,16.77 v61.99,17.27 | S1.3 51.96,34.17 v52.34,34.54 | S1.68 68.49,16.36 v67.83,17.02 | S1.25 52.14,23.17 v52.59,23.62 | S1.77 71.92,19.67 71.64,19.68 70.88,20.45 v70.88,20.7 | S1.49 58.99,17.06 v59.2,17.27 | S1.130 59.99,36.6 59.96,36.32 58.94,35.31 v58.69,35.31 | AVRUSB.S4 4.21,41.15 | C8.2 C9.2 6.53,24.55 v5.86,23.88 | 5.05,19.28 v5.88,20.12 6.62,19.38 C15.2 | C16.2 10.05,22.17 v10.02,22.2 | IC1.1 8.64,16.52 v8.4,16.76 | C17.2 v11.95,20.32 | U3.2 16.02,26.42 v16.27,26.67 | C18.2 15.34,23.2 v15.76,23.62 | C19.- 15.79,23.6 | 45.95,19.77 v44.97,18.8 | C4.2 46.21,35.34 v46.24,36.07 | 77.99,33.78 v77.99,35.05 | S1.73 71.25,17.67 v69.61,19.3 | C36.2 v71.14,12.19 | S1.108 73.54,35.17 v74.44,36.07 74.44,38.05 OSC.2@2 | v84.6,18.8 84.6,17.54 C26.2 | C35.2 63.77,44.07 v63.64,44.2
  Top 0.406: v57.42,42.93 C6.2 C7.2 | AVRUSB.P5 AVRUSB.S4 | SRAM.34 36.23,22.75 v36.34,22.86 | SRAM.12 35.43,30.1 v35.81,29.72
  Top 0.61: 14.51,45.1 13.75,45.99 13.75,49.8 C2.1 13.1,50.04 | 13.1,50.04 C1.1 | v13.1,52.45 13.1,50.04 | AVRUSB.S4 4.28,39.42 v4.59,39.12 | AVRUSB.S3 4.28,47.7 v4.59,48.01
  Route2 0.203: v46.24,36.07 45.23,36.07 | v35.83,46.23 35.83,45.97 | v28.46,12.45 28.72,12.45 | v34.81,12.45 34.56,12.45
  Route2 0.254: v34.05,27.18 34.05,27.69
  Bottom 0.203: U101.15 39.91,38.45 C105.2 | Y1.2 36.85,43.79 C107.2 36.45,45.61 v35.83,46.23 | 66,14.96 67.78,16.74 67.78,16.97 v67.83,17.02 | 65.16,7.88 v63.52,7.87 | 39.12,32.77 39.12,33.39 v39.64,33.91 | U101.5 33.27,32.77 32.77,33.27 32.13,33.27 C103.2
  Bottom 0.254: U101.33 43.41,30.77 42.91,31.27 | U101.5 39.12,32.77 | 39.12,32.77 39.13,32.77 | C102.1 34.8,27.93 v34.05,27.18 | U101.43 38.91,31.27 39.13,31.5 39.12,31.5 39.12,32.77
  Bottom 0.279: 39.91,34.27 U101.15 | U101.35 42.91,31.27
  Bottom 0.305: U101.EXP 39.91,34.27 | 42.91,31.27 U101.EXP | U101.EXP 43.15,35.51 43.3,35.51 43.56,35.77 U101.23 45.95,35.77 v46.24,36.07 | v71.14,12.19 71.28,12.05
  other vias: 13.1,51.44 6.87,29.84 2.68,34.54 2.68,30.73 1.67,32.77 1.29,45.72 1.29,41.4 2.68,43.56 1.29,48.39 1.16,38.73 42.18,33.91 40.91,33.91 11.95,43.18 12.97,43.18
  pour Bottom (isolate 0.305, rank 3): 0,56 100,56 100,0 0,0
  pour Route2: 0,56 100,56 100,0 0,0
  pour Top: -0.75,36.83 9.41,36.83 9.41,27.94 -0.75,27.94
  pour Top: -1,49.53 5.35,49.53 5.35,38.1 -1,38.1
  pour Top (no thermals): 11.45,46.23 17.03,46.23 17.03,42.42 11.45,42.42
MEGA_D0
  Top 0.203: S1.116 66.99,39.54 67.33,39.88 67.33,41.15 69.1,42.93 69.1,48.26 68.09,49.28 66.82,49.28 65.84,50.25 R21.1 65.08,50.25
MEGA_D1
  Top 0.203: S1.117 66.49,39.67 66.82,40.01 66.82,41.4 68.22,42.8 R20.1
MEGA_D2
  Top 0.203: S1.118 65.99,39.81 66.31,40.13 66.31,41.66 66.69,42.04 R19.1
MEGA_D3
  Top 0.203: S1.119 65.49,39.95 65.8,40.26 65.8,47.28 R18.1
MEGA_D4
  Top 0.203: R17.1 52.38,54.61 53.1,54.61 53.61,54.1 53.61,49.53 56.66,46.48 63.26,46.48 65.29,44.45 65.29,40.39 64.99,40.08 S1.120
MEGA_D5
  Top 0.203: R16.1 51.07,53.38 51.07,49.28 52.59,47.75 54.63,47.75 56.4,45.97 63.01,45.97 64.79,44.2 64.79,40.51 64.49,40.22 S1.121
MEGA_D6
  Top 0.203: S1.123 63.49,39.22 62.75,40.01 62.75,44.2 61.48,45.47 56.15,45.47 54.37,47.24 49.29,47.24 48.53,48.01 48.53,54.1 48.02,54.61 47.3,54.61 R15.1
MEGA_D7
  Top 0.203: S1.124 62.99,39.1 62.25,39.88 62.25,43.94 61.23,44.96 55.9,44.96 54.12,46.74 47.77,46.74 45.99,48.51 45.99,54.1 45.48,54.61 44.76,54.61 R14.1
MEGA_D8
  Top 0.203: S1.126 61.99,39.49 61.74,39.75 61.74,43.69 60.98,44.45 55.64,44.45 53.86,46.23 42.94,46.23 42.18,46.99 42.18,53.85 41.42,54.61 40.69,54.61 R13.1
MEGA_D9
  Top 0.203: S1.127 61.49,39.37 61.23,39.62 61.23,43.43 60.72,43.94 55.39,43.94 53.61,45.72 40.66,45.72 39.39,46.99 39.39,54.36 39.13,54.61 38.15,54.61 R12.1
MEGA_D10
  Top 0.203: S1.131 59.49,39.08 53.36,45.21 37.57,45.21 37.57,45.25 36.85,45.97 36.85,54.36 36.59,54.61 35.61,54.61 R11.1
MEGA_D11
  Top 0.203: S1.132 58.99,38.95 53.23,44.7 35.32,44.7 34.31,45.72 34.31,54.36 34.05,54.61 33.07,54.61 R10.1
MEGA_D12
  Top 0.203: S1.133 58.49,38.81 53.1,44.2 33.29,44.2 31.77,45.72 31.77,54.36 31.51,54.61 30.53,54.61 R9.1
MEGA_D13
  Top 0.203: S1.134 57.99,38.67 52.98,43.69 32.78,43.69 29.23,47.24 29.23,54.1 28.72,54.61 27.99,54.61 R8.1
MEGA_D14
  Top 0.203: S1.115 67.49,39.41 67.83,39.75 67.83,40.89 69.61,42.67 69.61,48.77 U1.D14
  Bottom 0.203: U101.30 52.1,32.27 54.63,34.8 54.63,45.97 57.17,48.51 65.29,48.51 U1.D14
MEGA_D15
  Top 0.203: S1.114 67.99,39.27 68.34,39.62 68.34,40.64 70.12,42.42 U1.D15
  Bottom 0.203: U101.31 52.36,31.77 55.13,34.54 55.13,45.72 57.42,48.01 67.33,48.01 U1.D15
MEGA_D16
  Top 0.203: S1.112 68.99,38.47 68.85,38.61 68.85,40.39 70.63,42.16 70.63,48.77 U1.D16
  Bottom 0.203: U101.32 52.63,31.27 55.64,34.29 55.64,45.47 57.67,47.5 69.36,47.5 U1.D16
MEGA_D17
  Top 0.203: S1.111 69.49,38.73 69.36,38.86 69.36,40.13 71.14,41.91 71.14,48.51 71.9,49.28 73.68,49.28 U1.D17
MEGA_D18
  Top 0.203: S1.105 73.81,33.67 76.47,36.32 79.52,36.32 80.03,36.83 80.03,44.7 77.74,46.99 U1.D18
MEGA_D19
  Top 0.203: U1.D19 82.82,48.26 82.82,36.83 78.76,32.77 75.2,32.77 74.6,32.17 S1.102
MEGA_D20
  Top 0.203: U1.D20 83.33,50.29 83.33,36.58 79.01,32.26 75.45,32.26 74.86,31.67 S1.101
MEGA_D21
  Top 0.203: U1.D21 83.84,49.28 83.84,36.32 79.26,31.75 75.71,31.75 75.12,31.17 S1.100
MEGA_D22
  Top 0.203: U1.D22 92.73,48.26 91.71,47.24 89.68,47.24 88.41,45.97 88.41,44.96 86.38,42.93 86.38,38.1 79.52,31.24 75.96,31.24 75.39,30.67 S1.99
MEGA_D23
  Top 0.203: U1.D23 94.76,48.26 93.49,46.99 92.22,46.99 91.96,46.74 89.93,46.74 88.92,45.72 88.92,44.7 86.88,42.67 86.88,37.85 79.77,30.73 76.22,30.73 75.65,30.17 S1.98
MEGA_D24
  Top 0.203: U1.D24 92.22,45.72 91.2,44.7 89.68,44.7 87.39,42.42 87.39,37.59 80.03,30.23 76.47,30.23 75.91,29.67 S1.97
MEGA_D25
  Top 0.203: U1.D25 94.76,45.72 93.49,44.45 92.22,44.45 91.96,44.2 89.93,44.2 87.9,42.16 87.9,37.34 80.28,29.72 76.72,29.72 76.22,29.21 74.69,29.21 74.15,28.67 S1.95
MEGA_D26
  Top 0.203: U1.D26 91.96,43.18 90.95,42.16 89.42,42.16 88.41,41.15 88.41,37.08 80.53,29.21 76.98,29.21 76.47,28.7 74.95,28.7 73.91,27.67 S1.93
MEGA_D27
  Top 0.203: U1.D27 94.76,43.18 93.49,41.91 92.22,41.91 91.96,41.66 89.68,41.66 88.92,40.89 88.92,36.83 80.79,28.7 77.23,28.7 76.72,28.19 75.2,28.19 74.17,27.17 S1.92
MEGA_D28/A5  (via drill 0.38)
  Top 0.203: S1.88 76.2,25.17 77.49,25.15 81.3,25.15 82.31,26.16 82.31,29.21 90.95,37.85 90.95,38.86 92.73,40.64 U1.D28
  Top 0.254: S1.88 68.62,25.17 68.09,24.64 60.21,24.64 v57.17,27.69
  Bottom 0.254: U101.36 42.41,22.88 42.94,22.35 48.78,22.35 53.86,27.69 v57.17,27.69 57.93,27.69 63.77,21.59 63.77,12.7 62.5,11.43 U1.A5
MEGA_D29
  Top 0.203: U1.D29 94.25,39.37 92.22,39.37 91.46,38.61 91.46,37.59 82.82,28.96 82.82,25.91 81.55,24.64 77.23,24.64 75.93,24.67 S1.87
MEGA_D30/A4  (via drill 0.38)
  Top 0.203: U1.D30 92.73,38.1 83.33,28.7 83.33,25.65 81.8,24.13 74.18,24.13 73.72,23.67 S1.85
  Top 0.254: v57.42,24.38 58.44,23.37 70.88,23.37 71.18,23.67 S1.85
  Bottom 0.254: U101.37 41.91,22.62 42.69,21.84 49.04,21.84 51.58,24.38 v57.42,24.38 59.96,24.38 63.26,21.08 63.26,12.95 61.74,11.43 61.74,4.32 U1.A4
MEGA_D31
  Top 0.203: U1.D31 94.25,36.83 92.22,36.83 83.84,28.45 83.84,25.4 82.06,23.62 74.44,23.62 73.98,23.17 S1.84
MEGA_D32/A3  (via drill 0.38)
  Top 0.203: U1.D32 91.71,35.56 84.34,28.19 84.34,25.15 82.31,23.11 74.69,23.11 74.24,22.67 S1.83
  Top 0.254: S1.83 57.73,22.67 v57.67,22.61
  Bottom 0.254: U101.38 41.41,22.11 42.18,21.34 51.58,21.34 52.85,22.61 v57.67,22.61 59.45,22.61 62.75,19.3 62.75,13.21 61.23,11.68 61.23,9.65 57.42,5.84 U1.A3
MEGA_D33
  Top 0.203: U1.D33 94.25,34.29 91.2,34.29 84.85,27.94 84.85,24.89 82.57,22.61 74.95,22.61 74.51,22.17 S1.82
MEGA_D34/A2  (via drill 0.38)
  Top 0.203: U1.D34 90.69,33.02 85.36,27.69 85.36,24.64 82.82,22.1 75.2,22.1 74.77,21.67 S1.81
  Top 0.254: S1.81 59.27,21.67 v58.44,20.83
  Bottom 0.254: U101.39 40.91,21.84 41.93,20.83 v58.44,20.83 60.72,18.54 60.72,9.91 57.17,6.35 56.15,6.35 54.88,5.08 U1.A2
MEGA_D35
  Top 0.203: U1.D35 94.25,31.75 90.19,31.75 85.87,27.43 85.87,24.38 83.07,21.59 75.45,21.59 75.03,21.17 S1.80
MEGA_D36
  Top 0.203: U1.D36 89.68,30.48 86.38,27.18 86.38,24.13 83.33,21.08 75.71,21.08 75.29,20.67 S1.79
MEGA_D37
  Top 0.203: U1.D37 94.25,29.21 89.17,29.21 86.88,26.92 86.88,23.88 83.58,20.57 75.96,20.57 75.55,20.17 S1.78
MEGA_D38
  Top 0.203: S1.75 74.31,18.67 74.56,18.67 82.44,18.67 87.39,23.62 87.39,25.4 88.92,26.92 91.96,26.92 U1.D38
MEGA_D39
  Top 0.203: S1.74 74.05,18.17 74.31,18.16 82.69,18.16 87.9,23.37 87.9,25.15 89.17,26.42 92.22,26.42 92.47,26.67 94.25,26.67 U1.D39
MEGA_D40
  Top 0.203: U1.D40 92.98,24.89 92.73,24.64 91.71,24.64 91.46,24.38 89.68,24.38 87.9,22.61 87.9,17.02 83.58,12.7 73.17,12.7 72.28,13.59 68.72,13.59 67.99,14.32 S1.67
MEGA_D41
  Top 0.203: S1.66 67.49,14.06 68.47,13.08 72.03,13.08 72.91,12.19 83.84,12.19 88.41,16.76 88.41,22.35 89.93,23.88 91.71,23.88 91.96,24.13 94.25,24.13 U1.D41
MEGA_D42
  Top 0.203: S1.62 65.49,12.25 66.31,11.43 71.64,11.43 71.9,11.68 84.09,11.68 88.92,16.51 88.92,20.57 89.93,21.59 91.2,21.59 92.47,22.86 U1.D42
MEGA_D43
  Top 0.203: S1.61 64.99,12.12 66.18,10.92 71.9,10.92 72.15,11.18 84.34,11.18 89.42,16.26 89.42,17.53 91.71,19.81 91.71,21.08 92.22,21.59 94.25,21.59 U1.D43
MEGA_D44
  Top 0.203: U1.D44 89.93,17.27 89.93,16 84.6,10.67 72.41,10.67 72.15,10.41 66.06,10.41 63.99,12.48 S1.59
MEGA_D45
  Top 0.203: U1.D45 94.76,20.32 93.49,19.05 92.47,19.05 90.44,17.02 90.44,15.75 84.85,10.16 72.66,10.16 72.41,9.91 65.93,9.91 63.49,12.35 S1.58
MEGA_D46
  Top 0.203: U1.D46 92.22,17.78 90.95,16.51 90.95,15.49 85.11,9.65 72.91,9.65 72.66,9.4 65.8,9.4 62.99,12.21 S1.57
MEGA_D47
  Top 0.203: U1.D47 94.76,17.78 93.49,16.51 92.22,16.51 91.46,15.75 91.46,15.24 85.36,9.14 73.17,9.14 72.91,8.89 65.67,8.89 62.49,12.08 S1.56
MEGA_D48
  Top 0.203: U1.D48 92.22,15.24 83.33,6.35 69.36,6.35 67.33,8.38 65.55,8.38 61.99,11.94 S1.55
MEGA_D49
  Top 0.203: U1.D49 94.76,15.24 93.49,13.97 91.71,13.97 83.58,5.84 69.1,5.84 68.09,6.86 60.21,6.86 58.94,8.13 58.94,11.94 59.99,12.98 S1.51
MEGA_D50
  Top 0.203: U1.D50 91.2,12.7 83.84,5.33 68.85,5.33 67.83,6.35 59.96,6.35 58.44,7.87 58.44,12.19 59.49,13.24 S1.50
MEGA_D51
  Top 0.203: U1.D51 94.76,12.7 93.49,11.43 90.69,11.43 84.09,4.83 68.6,4.83 67.58,5.84 59.71,5.84 57.93,7.62 57.93,12.45 58.49,13.01 S1.48
MEGA_D52
  Top 0.203: U1.D52 90.19,10.16 84.34,4.32 68.34,4.32 67.33,5.33 59.45,5.33 57.42,7.37 57.42,12.7 57.99,13.27 S1.47
MEGA_D53  (via drill 0.38)
  Top 0.203: v51.07,9.65 R32.1 52.59,9.61 52.59,8.89 56.66,4.83 66.56,4.83 67.07,4.32 67.07,4.3 67.56,3.81 85.34,3.81 90.42,8.89 94.25,8.89 U1.D53
  Top 0.305: S1.39 53.99,17.4 v54.63,18.03
  Bottom 0.203: v54.63,18.03 52.09,18.03 50.31,16.26 50.31,10.41 v51.07,9.65
N$2
  Top 0.203: LED.A 24.56,42.26 24.15,42.67 24.15,51.78 R7.1
N$8
  Top 0.203: PWR.A 20.09,54.14 R6.1
N$9
  Top 0.203: IC1.6 6.35,13.31 R27.2
N$22
  Top 0.178: C9.1 8.23,22.69 X1.1
  Top 0.203: IC1.2 9.49,15.31 9.67,15.49 9.67,17.78 8.4,19.05 8.4,22.35 X1.1
N$23
  Top 0.178: C8.1 3.1,22.64 X1.2
  Top 0.203: IC1.3 7.81,14.81 7.64,14.99 7.64,19.56 6.11,21.08 4.59,21.08 X1.2
N$24
  Top 0.305: R30.2 RX.C
N$25
  Top 0.305: R29.2 TX.C
N$45
  Top 0.203: R25.1 R26.1 17.07,31.08 17.29,30.86 17.29,26.42 16.4,25.53 15.09,25.53 U3.1
N$48
  Top 0.203: L3.1 3.81,16.93 C14.+ 5.11,16.93 C15.1 6.37,16.68 6.37,14.73 6.78,14.31 IC1.4
N$49
  Top 0.203: IC1.9 3.07,11.81 2.43,11.18 2.43,7.37 3.83,5.97 L4.1
  Top 0.254: C34.1 7.42,3.16 C28.+ 6.15,4.43 L4.1
OSC_IN
  Top 0.203: OSC.3@3 77.64,38.2 76.22,39.62 72.91,39.62 71.39,38.1 71.39,36.32 70.88,35.81 69.61,35.81 68.6,34.8 68.6,30.23 70.66,28.17 S1.94
RESET  (via drill 0.38)
  Top 0.203: SW2.A 28.08,9.91 26.18,9.91 25.16,8.89 25.16,6.1 26.04,5.22 R31.1 26.92,5.21 26.92,2.79 28.7,1.02 32.26,1.02 33.27,2.03 33.27,4.32 v34.91,5.96 SW2.A'
  Top 0.305: S1.37 52.16,15.32 v52.09,15.24
  Bottom 0.203: v52.09,15.24 58.18,15.24 58.69,14.73 58.69,10.16 56.4,7.87 51.32,7.87 49.29,5.84 35.03,5.84 v34.91,5.96
SW1
  Top 0.203: S1.104 74.08,33.17 76.72,35.81 79.77,35.81 80.53,36.58 80.53,40.39 SW1.COM2
SW_1V2
  Top 0.254: U2.8 19.15,46.99 L2.1
SW_3V3
  Top 0.254: U2.4 11.33,46.49 11.19,46.35 11.19,44.2 10.43,43.43 9.24,43.43 L1.1
UCAP
  Bottom 0.203: U101.6 33.78,33.27 32.77,34.29 30.73,34.29 30.48,34.04 30.48,33.4 C103.1
XTAL1
  Bottom 0.203: C107.1 34.7,42.35 Y1.1 | 34.81,44.31 C107.1 | U101.17 40.91,41.15 39.39,42.67 39.01,42.67 R109.1 38.88,44.96 36.59,47.24 35.32,47.24 34.56,46.48 34.56,44.34 C107.1
XTAL2
  Bottom 0.203: C106.2 36.45,39.95 Y1.3 36.85,40.65 37.35,41.15 38.75,41.15 R109.2 39.01,41.15 39.89,41.15 40.41,40.63 U101.16
  Bottom 0.305: Y1.3 36.72,40.35

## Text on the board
tNames: GND | 3.3V | 5V | GND | 3.3V | 5V
bNames: U11
tDocu: Top silkscreen is on layer 130: tSilk | Bottom silkscreen is on layer 200
tSilk: AVR USB | AL | BL | AVR | GND | 5V | FPGA USB | FPGA | CL | JTAG | C | DH | D | 6/4/2014 | CH | DL | FPGA Reset | Papilio Platform | Papilio Duo | www.GadgetFactory.net | www.Papilio.cc | BPC3013 V1.4 | CC-BY-SA 4.0 | Copyright 2014 | Gadget Factory, LLC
